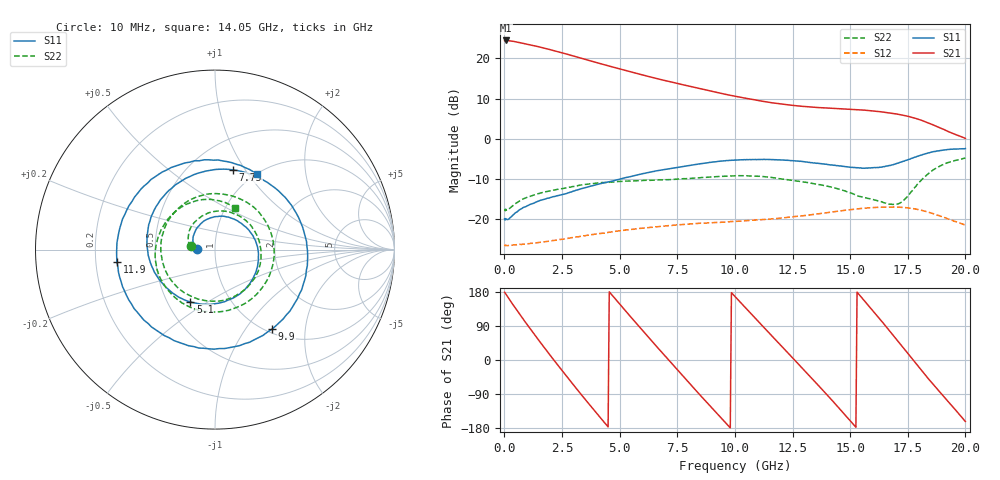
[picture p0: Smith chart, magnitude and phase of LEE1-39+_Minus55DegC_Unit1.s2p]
!Keysight Technologies,N5245A,MY52442000,A.10.65.23
!Date: Tuesday, November 25, 2025 21:47:15
!Correction: S11(Full 2 Port(1,2))
!S21(Full 2 Port(1,2))
!S12(Full 2 Port(1,2))
!S22(Full 2 Port(1,2))
!S2P File: Measurements: S11, S21, S12, S22:
!Deduct Board Loss
# Hz S  dB  R 50
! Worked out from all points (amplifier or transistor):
!   408 points, 10 MHz to 20 GHz, reference 50 ohm
!   highest |S21| = 24.5 dB at 80 MHz (marker M1)
!   |S21| within 3 dB of that: start of sweep to 2.455 GHz
!   unconditionally stable (mu >= 1): start of sweep to end of sweep
!   at 3.05 GHz: K = 1.05, MAG = 21.1 dB, |S12| = -24.4 dB
!   at 9.85 GHz: K = 1.23, MAG = 12.8 dB, |S12| = -20.5 dB
!   at 20 GHz: K = 1.86, MAG = 5.4 dB, |S12| = -21.4 dB
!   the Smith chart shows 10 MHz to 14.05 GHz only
!   S11 on the Smith chart (normalised r, x): 10 MHz: 0.81, +0.01; 5.1 GHz: 0.65, -0.42; 7.75 GHz: 0.79, +0.88; 9.9 GHz: 1.06, -1.34; 11.9 GHz: 0.29, -0.06; 14.05 GHz: 1.01, +1.10
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1e7  -19.79 177.8  24.41 178.8  -26.63 1.9  -17.38 170.8
8e7  -19.88 -179.8  24.47 172.6  -26.41 -3.4  -17.69 177.7
5e8  -18.27 166.0  24.12 134.9  -26.31 -23.5  -15.99 159.9
9e8  -16.87 145.4  23.66 100.8  -26.09 -42.9  -14.68 135.1
1.3e9  -15.90 122.9  23.15 67.7  -25.84 -63.3  -13.90 108.4
1.85e9  -14.75 91.2  22.38 23.3  -25.46 -91.3  -13.06 71.8
2.7e9  -13.55 38.5  21.09 -43.1  -24.70 -135.6  -12.12 16.6
3.35e9  -12.33 -3.1  20.02 -92.3  -24.17 -170.9  -11.39 -26.9
4.2e9  -11.07 -57.2  18.65 -154.8  -23.46 142.3  -10.85 -82.6
5.1e9  -9.83 -115.1  17.26 140.6  -22.72 90.8  -10.54 -141.3
5.85e9  -8.84 -162.7  16.12 87.9  -22.22 47.7  -10.35 168.8
6.7e9  -7.82 143.9  14.88 29.1  -21.75 -1.9  -10.17 112.0
7.75e9  -6.83 77.4  13.47 -42.6  -21.24 -63.5  -9.88 43.2
8.65e9  -6.04 20.7  12.28 -103.2  -20.90 -116.8  -9.55 -13.7
9.9e9  -5.27 -54.5  10.74 174.4  -20.51 170.5  -9.18 -88.9
1.005e10  -5.24 -63.4  10.57 164.6  -20.47 161.8  -9.16 -97.4
1.19e10  -5.19 -172.7  8.75 44.6  -19.71 54.3  -9.83 165.3
1.335e10  -5.88 103.0  7.92 -49.3  -18.78 -31.1  -11.01 95.9
1.405e10  -6.38 60.8  7.67 -95.3  -18.26 -73.1  -11.78 65.0
1.535e10  -7.14 -26.6  7.27 175.5  -17.36 -155.0  -14.19 -5.2
1.67e10  -6.59 -134.6  6.48 77.8  -16.91 114.4  -16.19 -116.7
2e10  -2.39 -6.3  0.12 -162.2  -21.43 -107.7  -4.74 -17.8
